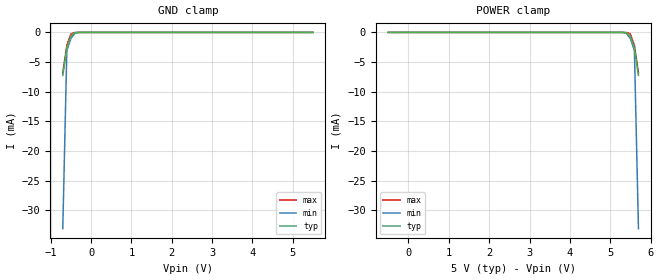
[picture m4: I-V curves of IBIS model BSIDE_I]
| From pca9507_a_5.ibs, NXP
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[Model]   BSIDE_I
Model_type Input
Vinh=3.5
Vinl=1.5
C_comp   4.8p   4.6p   5p
[Temperature Range] 27   85   -40
[Voltage Range]   5   4.5   5.5
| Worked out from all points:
|   GND clamp passes 1 mA (typ) near -0.52 V on its own axis
[GND Clamp]
-700mV    -7.261mA   -33.13mA   -6.825mA
-600mV    -2.645mA   -3.106mA   -2.2mA
-500mV    -659.2uA   -1.029mA   -279.4uA
-400mV    -54.1uA    -160uA     -7.518uA
-200mV    -25.23nA   -194.8nA   -665.6pA
5.5V      352.9pA    608.6pA    327.7pA
[POWER Clamp]
-500mV    352.9pA    608.6pA    327.7pA
5.2V      -25.23nA   -194.8nA   -665.6pA
5.4V      -54.1uA    -160uA     -7.518uA
5.5V      -659.2uA   -1.029mA   -279.4uA
5.6V      -2.645mA   -3.106mA   -2.2mA
5.7V      -7.261mA   -33.13mA   -6.825mA
